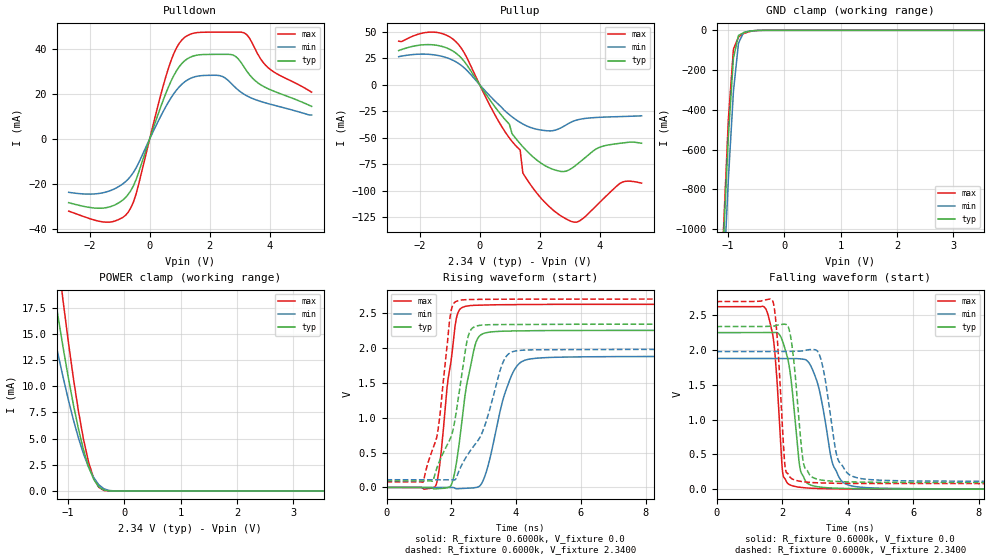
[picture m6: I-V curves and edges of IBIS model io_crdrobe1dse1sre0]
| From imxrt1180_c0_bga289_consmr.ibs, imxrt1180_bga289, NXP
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[Model]  io_crdrobe1dse1sre0
|   Model io_crdrobe1dse1sre0
| This model was characterised for following simulation conditions:
| External (pad) voltage:
|   - Typ: 2.34V,   - Min: 1.98V,   - Max: 2.7V
| Library cells for typ/min/max conditions are connected as defined below:
|  PAD_IO - External Pad
|  ipp_do - Core Input
|  ipp_obe - Output Buffer Enable
|  ASRCN3V3[3] - NC
|  ASRCN3V3[4] - NC
|  ASRCP3V3[4] - NC
|  REFAPBIAS3V3 - gnde
|  REFBAMPL3V3 - vdd1v8
|  REFCAMPH3V3 - vdd1v8
|  REFDNBIAS3V3 - vdd1v8
|  REFH3V3 - REFH3V3
|  REFL3V3 - REFL3V3
|  gnde - gnde
|  ipp_dse - vdd
|  ipp_ina235_3v - NC
|  ipp_ina40_3v - NC
|  ipp_ina_mux - NC
|  ipp_ind - NC
|  ipp_ind_1p8v - NC
|  ipp_ind_3v - NC
|  ipp_sre - gnde
|  vdd - vdd
|  vdd1v8 - vdd1v8
|  vdda - vdde3v3
|  vdde3v3 - vdde3v3
| All other pins connected to ground
Model_type I/O
Polarity   Non-Inverting
Enable   Active-High
Vinl =   0.7020V
Vinh =   1.6300V
Vmeas =  1.1700V
Cref =   15.0000pF
Rref =   0.6000k
Vref =   0.0V
C_comp   3.9951pF   3.8194pF   4.1033pF
|C_comp_pullup   0.5141pF   0.5881pF   0.4995pF
|C_comp_pulldown   2.0717pF   2.1609pF   1.8544pF
[Model Spec]
| variable   typ   min   max
Vinh   1.6300V   NA   NA
Vinl   0.7020V   NA   NA
Vref   0.0V   0.0V   0.0V
Cref   15.0000pF   15.0000pF   15.0000pF
Rref   0.6000k   0.6000k   0.6000k
[Receiver Thresholds]
Vcross_high  =   0.0V
Vcross_low  =   0.0V
Vdiff_ac  =   0.0V
Vdiff_dc  =   0.0V
Tdiffslew_ac  =   0.0S
[Temperature Range]   25.0000   0.1250k   -40.0000
[Voltage Range]   2.3400V   1.9800V   2.7000V
[Pullup Reference]   2.3400V   1.9800V   2.7000V
[Pulldown Reference]   0.0V   0.0V   0.0V
[POWER Clamp Reference]   2.3400V   1.9800V   2.7000V
[GND Clamp Reference]   0.0V   0.0V   0.0V
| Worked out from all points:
|   slope of the pulldown table from 0 to 0.351 V, typ, clamps not added: 25.9 ohm
|   slope of the pullup table from 0 to 0.351 V, typ, clamps not added: 23.9 ohm
|   GND clamp passes 1 mA (typ) near -0.49 V on its own axis
|   POWER clamp passes 1 mA (typ) near -0.53 V on its own axis
|   rising waveform, R_fixture 0.6000k, V_fixture 0.0: 20-80 % time 433ps typ, 603ps min, 371ps max; typ from 0 V to 2.25 V
|   rising waveform, R_fixture 0.6000k, V_fixture 2.3400: 20-80 % time 609ps typ, 937ps min, 429ps max; typ from 0.094 V to 2.34 V
|   falling waveform, R_fixture 0.6000k, V_fixture 0.0: 20-80 % time 299ps typ, 442ps min, 223ps max; typ from 2.25 V to 0 V
|   falling waveform, R_fixture 0.6000k, V_fixture 2.3400: 20-80 % time 254ps typ, 362ps min, 194ps max; typ from 2.34 V to 0.094 V
[Pulldown]
|Voltage   I(typ)   I(min)   I(max)
-2.7V     -28.24mA   -23.65mA   -31.99mA
-1.44V    -30.44mA   -23.46mA   -36.9mA
-720mV    -24.64mA   -17.86mA   -32.55mA
-450mV    -17.94mA   -12.78mA   -24.31mA
630mV     23.17mA    16.47mA    31.53mA
900mV     30.36mA    21.79mA    40.52mA
1.26V     35.6mA     26.18mA    45.89mA
2.34V     37.55mA    28.09mA    47.4mA
2.79V     37.18mA    23.72mA    47.41mA
3.15V     31.9mA     19.83mA    47.08mA
3.96V     22.22mA    15.65mA    31.51mA
5.4V      14.48mA    10.63mA    20.78mA
[Pullup]
|Voltage   I(typ)   I(min)   I(max)
-2.7V     32.17mA    26.42mA    41.08mA
-1.53V    37.55mA    28.2mA     49.59mA
-720mV    28.16mA    20.36mA    38.44mA
630mV     -25.37mA   -18.65mA   -34.47mA
1.35V     -55.63mA   -35.58mA   -61.51mA
1.44V     -58.52mA   -37.05mA   -83.28mA
2.16V     -76.03mA   -43.22mA   -110.5mA
2.88V     -81.56mA   -38mA      -126.6mA
3.33V     -73.2mA    -32.68mA   -128.5mA
4.05V     -58.5mA    -30.69mA   -109.7mA
4.77V     -54.96mA   -30mA      -91.76mA
5.4V      -55.22mA   -29.38mA   -92.86mA
[GND_clamp]
|Voltage   I(typ)   I(min)   I(max)
-2.7V     -12.91A    -12.88A    -13.56A
-1.08V    -1.077A    -1.286A    -1.025A
-990mV    -533.6mA   -749.4mA   -449.1mA
-900mV    -139.2mA   -307mA     -94.25mA
-810mV    -25.49mA   -63.91mA   -32.87mA
-720mV    -11.78mA   -11.41mA   -16.65mA
-540mV    -1.684mA   -1.901mA   -2.149mA
-360mV    -36.04uA   -133.3uA   -15.05uA
5.4V      0A         0A         0A
[POWER_clamp]
|Voltage   I(typ)   I(min)   I(max)
-2.7V     73.96mA    57.58mA    95.4mA
-1.44V    26.15mA    20.18mA    34.67mA
-1.35V    22.86mA    17.7mA     30.34mA
-1.26V    19.66mA    15.3mA     26.09mA
-1.17V    16.56mA    12.98mA    21.97mA
-1.08V    13.59mA    10.78mA    17.99mA
-900mV    8.212mA    6.776mA    10.73mA
-720mV    3.9mA      3.518mA    4.888mA
-630mV    2.284mA    2.252mA    2.724mA
-540mV    1.103mA    1.268mA    1.195mA
-360mV    77.93uA    204.3uA    41.52uA
5.4V      0A         0A         0A
[Ramp]
| variable   typ   min   max
dV/dt_r  1.3518/0.4325n   1.1288/0.6031n   1.5754/0.3710n
dV/dt_f  1.3475/0.2543n   1.1218/0.3619n   1.5719/0.1936n
R_load = 0.6000k
[Rising Waveform]
R_fixture= 0.6000k
V_fixture= 0.0
V_fixture_min= 0.0
V_fixture_max= 0.0
|time   V(typ)   V(min)   V(max)
0s        54.47nV    1.425uV    18.12nV
1.52ns    -19.95mV   -587.2uV   25.41mV
1.659ns   -16.62mV   -640.1uV   386.8mV
1.97ns    15.45mV    -238.9uV   1.748V
2.151ns   331.3mV    -19.15mV   2.411V
2.632ns   1.822V     -8.959mV   2.608V
3.023ns   2.211V     143.2mV    2.615V
3.898ns   2.243V     1.643V     2.621V
4.695ns   2.248V     1.855V     2.623V
60ns      2.253V     1.881V     2.626V
[Rising Waveform]
R_fixture= 0.6000k
V_fixture= 2.3400
V_fixture_min= 1.9800
V_fixture_max= 2.7000
|time   V(typ)   V(min)   V(max)
0s        94.13mV    110.3mV    80.1mV
1.136ns   93.6mV     110.2mV    81.32mV
1.587ns   320.4mV    109.7mV    811.2mV
1.998ns   733.1mV    110.4mV    2.539V
2.375ns   1.781V     368.3mV    2.689V
2.695ns   2.299V     593.3mV    2.695V
3.023ns   2.33V      870.6mV    2.696V
3.648ns   2.335V     1.842V     2.698V
4.229ns   2.337V     1.968V     2.699V
60ns      2.34V      1.98V      2.7V
[Falling Waveform]
R_fixture= 0.6000k
V_fixture= 0.0
V_fixture_min= 0.0
V_fixture_max= 0.0
|time   V(typ)   V(min)   V(max)
0s        2.253V     1.881V     2.626V
1.514ns   2.254V     1.881V     2.582V
1.756ns   2.253V     1.881V     2.075V
1.94ns    2.209V     1.881V     795.5mV
2.043ns   2.088V     1.882V     177.9mV
2.668ns   159mV      1.87V      20.43mV
3.083ns   34.54mV    1.521V     9.512mV
3.59ns    15.01mV    309.7mV    4.394mV
4.508ns   5.769mV    23.98mV    1.348mV
60ns      1.226uV    6.671uV    687.5nV
[Falling Waveform]
R_fixture= 0.6000k
V_fixture= 2.3400
V_fixture_min= 1.9800
V_fixture_max= 2.7000
|time   V(typ)   V(min)   V(max)
0s        2.34V      1.98V      2.7V
1.717ns   2.344V     1.98V      2.704V
1.85ns    2.36V      1.979V     2.183V
2.078ns   2.374V     1.981V     375.5mV
2.174ns   2.348V     1.982V     224.8mV
2.762ns   271.8mV    2.004V     100.5mV
3.189ns   132mV      1.858V     89.27mV
3.739ns   109.2mV    390.9mV    84mV
4.77ns    99.15mV    134.4mV    81.13mV
60ns      94.14mV    110.3mV    80.1mV
